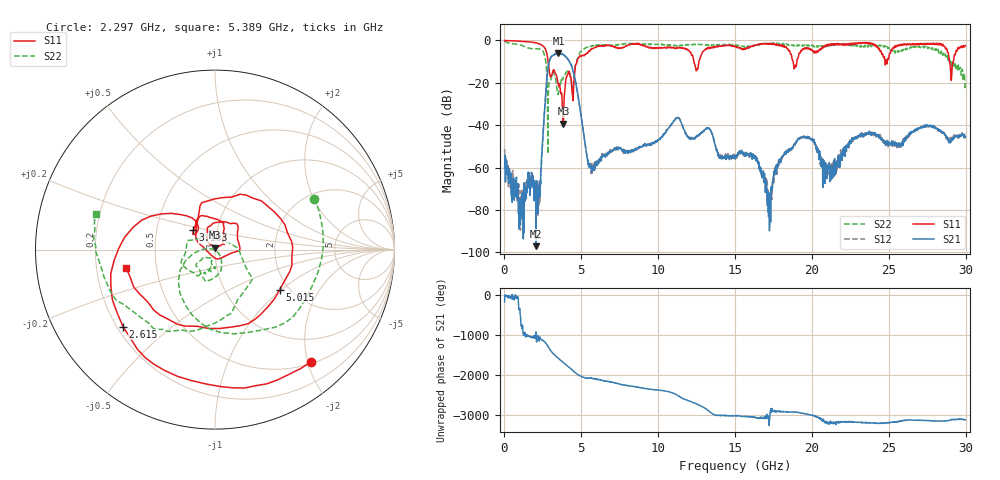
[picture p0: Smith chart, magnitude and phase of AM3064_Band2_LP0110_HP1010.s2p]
# Hz S DB R 50.0
!freq dBS11 angS11 dBS21 angS21 dBS12 angS12 dBS22 angS22
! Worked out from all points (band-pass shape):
!   1600 points, 10 MHz to 29.98 GHz, reference 50 ohm
!   highest |S21| = -6.08 dB at 3.515 GHz (marker M1); lowest = -97.1 dB at 2.053 GHz (marker M2)
!   |S21| within 3 dB of the highest: 2.951 GHz to 4.146 GHz (1.195 GHz wide, 33.7 % of centre)
!   lowest |S11| = -39.3 dB at 3.834 GHz (marker M3), VSWR 1.02, Z = 50.2 + j1.06 ohm
!   |S11| at or under -10 dB: 2.84 GHz to 4.72 GHz (1.88 GHz wide, 49.7 % of centre); 12.32 GHz to 12.65 GHz (327.9 MHz wide, 2.63 % of centre); 28.95 GHz to 29.2 GHz (255.5 MHz wide, 0.879 % of centre)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
!   |S22| runs from -53.5 to -0.3 dB; largest |S21 - S12| = 0.018
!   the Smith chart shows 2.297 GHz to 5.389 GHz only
!   S11 on the Smith chart (normalised r, x): 2.297 GHz: 0.53, -2.06; 2.615 GHz: 0.22, -0.35; 3.103 GHz: 0.77, +0.17; 5.015 GHz: 1.79, -0.97; 5.389 GHz: 0.33, -0.09
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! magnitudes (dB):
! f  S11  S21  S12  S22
! 10 MHz  0.0  -60.2  -51.2  -0.3
! 1.041 GHz  -0.4  -84.7  -89.6  -2.2
! 2.053 GHz  -1.2  -97.1  -69.0  -3.8
! 2.297 GHz  -1.7  -70.2  -75.2  -4.1
! 2.615 GHz  -3.5  -32.3  -32.2  -7.1
! 2.878 GHz  -12.2  -11.1  -11.1  -21.8
! 3.103 GHz  -15.8  -7.4  -7.3  -16.3
! 3.515 GHz  -20.9  -6.1  -6.1  -25.1
! 3.834 GHz  -39.3  -6.8  -6.7  -17.1
! 5.015 GHz  -7.4  -37.2  -37.0  -5.0
! 5.389 GHz  -5.9  -55.3  -55.7  -3.2
! 10 GHz  -3.6  -47.2  -47.3  -1.9
! 11.27 GHz  -3.5  -36.4  -36.3  -2.6
! 15 GHz  -2.7  -55.7  -55.0  -2.0
! 16.3 GHz  -2.2  -54.5  -54.9  -2.2
! 17.22 GHz  -1.3  -83.9  -81.1  -1.6
! 18.14 GHz  -3.1  -54.3  -54.5  -1.9
! 19.99 GHz  -4.5  -46.3  -46.9  -2.2
! 21.25 GHz  -1.6  -64.4  -60.6  -2.4
! 23.1 GHz  -1.4  -45.2  -45.0  -2.4
! 25 GHz  -8.4  -49.5  -49.1  -3.3
! 29.98 GHz  -2.4  -45.6  -45.8  -20.3
